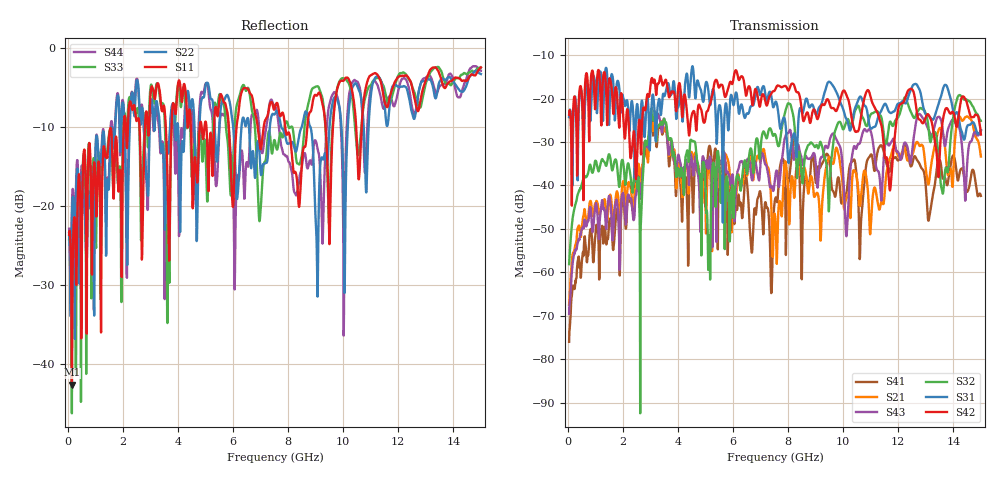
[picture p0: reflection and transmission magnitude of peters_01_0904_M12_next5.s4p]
# MHZ S RI R 50.00
! FREQ  S11  S12  S13  S14
!  S21  S22  S23  S24
!  S31  S32  S33  S34
!  S41  S42  S43  S44
!  REAL  IMAG  REAL  IMAG  REAL  IMAG  REAL  IMAG
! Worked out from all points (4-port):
!   1496 points, 50 MHz to 15 GHz, reference 50 ohm
!   strongest paths, dB at 50 MHz, 3.79 GHz, 7.53 GHz, 11.27 GHz, 15 GHz:
!     S42: -23.7, -18.5, -18.0, -23.6, -28.3
!     S31: -24.3, -18.6, -20.9, -24.2, -27.2
!     S32: -58.1, -31.2, -28.2, -23.1, -25.1
!     S43: -69.6, -30.1, -38.2, -36.7, -27.4
!     S21: -67.4, -31.3, -47.2, -44.5, -33.3
!     S41: -76.0, -31.3, -43.2, -31.7, -42.4
!   lowest |S11| = -42.6 dB at 150 MHz (marker M1), VSWR 1.01, Z = 49.4 + j0.478 ohm
!   |S11| at or under -10 dB: start of sweep to 2.031 GHz; 4.472 GHz to 4.789 GHz (317.4 MHz wide, 6.85 % of centre); 7.897 GHz to 8.695 GHz (797.9 MHz wide, 9.62 % of centre)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
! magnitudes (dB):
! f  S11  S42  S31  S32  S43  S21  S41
! 50 MHz  -23.6  -23.7  -24.3  -58.1  -69.6  -67.4  -76.0
! 150 MHz  -42.6  -44.7  -32.9  -49.1  -60.0  -57.4  -65.3
! 3.11 GHz  -5.3  -16.4  -19.7  -25.2  -24.9  -27.3  -28.2
! 5.12 GHz  -17.1  -22.0  -19.0  -53.4  -35.8  -35.7  -31.4
! 8.02 GHz  -10.6  -18.1  -34.9  -21.1  -27.9  -45.4  -39.2
! 10.12 GHz  -3.7  -19.2  -24.7  -25.2  -51.7  -43.0  -41.6
! 15 GHz  -2.4  -28.3  -27.2  -25.1  -27.4  -33.3  -42.4
